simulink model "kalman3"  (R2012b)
settings: Solver=ode45  StartTime=0.0  StopTime=50.0  RelTol=1e-3
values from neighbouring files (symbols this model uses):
  A1 = 0.02    [fuellstnd_1.m]    (also in fuellstnd_2.m; fuellstnd_21.m; fuellstnd_3.m; fuellstnd_31.m)
  A2 = A1    (= 0.02)    [fuellstnd_1.m]    (also in fuellstnd_2.m; fuellstnd_21.m; fuellstnd_3.m; fuellstnd_31.m)
  B1 = sys1.b    [kalman_11.m]    (also in kalman_12.m; kalman_13.m; kalman_2.m; kalman_3.m)
  B2 = sys2.b    [kalman_2.m]    (also in kalman_3.m)
  C1 = sys1.c    [kalman_11.m]    (also in kalman_12.m; kalman_13.m; kalman_2.m; kalman_3.m)
  C2 = sys2.c    [kalman_2.m]    (also in kalman_3.m; feder_masse_1.m = [0 0 1 0]; feder_masse_13.m = [0 0 1 0]; feder_masse_14.m = [0 0 1 0])
  dt = 0.01    [aktiv_tilger_1.m]    (also in aktiv_tilger_12.m; aktiv_tilger_2.m; beobachter_1.m; beobachter_2.m)
  Kest = kalman(P,1,0.01),    [LQG_1.m]    (also in ss_zwei_eing_1.m = kalman(sys2, Q, R))
  ki = -Kn(n+1)    [beobachter_2.m]    (also in beobachter_22.m; kalman_12.m = -Kn(3); kalman_13.m = -Kn(4); kalman_d1.m = -Kn(4))
  Kr = 2000    [aktiv_tilger_2.m]    (also in beobachter_22.m = 5; fuellstnd_3.m = 10,; fuellstnd_31.m = 10,; kalman_12.m = Kn(1:2))
  vnd = 1e-4    (= 0.0001)    [kalman_1.m]    (also in kalman_10.m; kalman_11.m; kalman_12.m; kalman_13.m = 0.01)
  vny = 1e-6    (= 1e-06)    [kalman_1.m]    (also in kalman_10.m; kalman_11.m = ', num2str(vny),' )']); kalman_12.m = ', num2str(vny),' )']); kalman_13.m = ', num2str(vny),' )']))

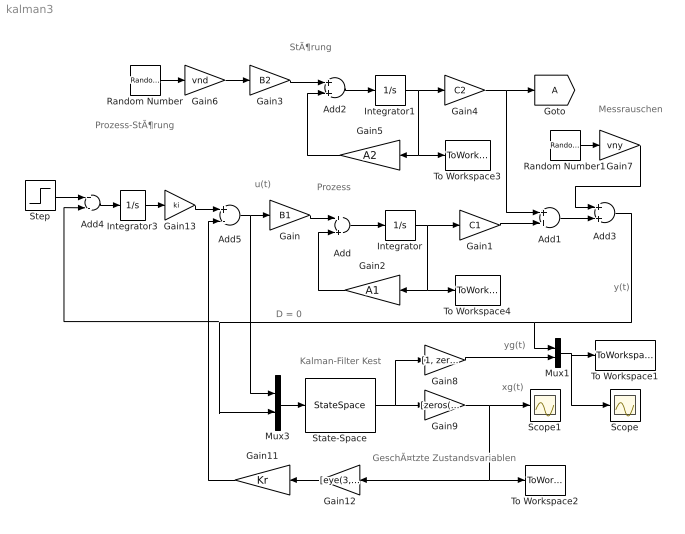
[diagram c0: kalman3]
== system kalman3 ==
  note: StÃ¶rung
  note: Prozess
  note: Prozess-StÃ¶rung
  note: Messrauschen
  note: xg(t)
  note: y(t)
  note: u(t)
  note: D = 0
  note: Kalman-Filter Kest
  note: yg(t)
  note: GeschÃ¤tzte Zustandsvariablen
  Add{,1..3} (4 alike) : Sum
  Add4 : Sum  Inputs=+-
  Add5 : Sum  Inputs=+-
  Gain : Gain  Gain=B1  Multiplication=Matrix(K*u)
  Gain1 : Gain  Gain=C1  Multiplication=Matrix(K*u)
  Gain11 : Gain  Gain=Kr  Multiplication=Matrix(K*u)
  Gain12 : Gain  Gain=[eye(3,3), zeros(3,3)]  Multiplication=Matrix(K*u)
  Gain13 : Gain  Gain=ki
  Gain2 : Gain  Gain=A1  Multiplication=Matrix(K*u)
  Gain3 : Gain  Gain=B2  Multiplication=Matrix(K*u)
  Gain4 : Gain  Gain=C2  Multiplication=Matrix(K*u)
  Gain5 : Gain  Gain=A2  Multiplication=Matrix(K*u)
  Gain6 : Gain  Gain=vnd
  Gain7 : Gain  Gain=vny
  Gain8 : Gain  Gain=[1, zeros(1,6)]  Multiplication=Matrix(K*u)
  Gain9 : Gain  Gain=[zeros(6,1),eye(6,6)]  Multiplication=Matrix(K*u)
  Integrator : Integrator
  Integrator1 : Integrator
  Integrator3 : Integrator
  Mux1 : Mux  Inputs=2
  Mux3 : Mux  Inputs=2
  Random Number : RandomNumber  SampleTime=dt*10
  Random Number1 : RandomNumber  Seed=18967  SampleTime=dt*10
  Scope : Scope
  Scope1 : Scope
  State-Space : StateSpace  A=Kest.a  B=Kest.b  C=Kest.c  D=Kest.d
  Step : Step  SampleTime=0
  To Workspace1 : ToWorkspace  VariableName=y1  SaveFormat=Structure With Time
  To Workspace2 : ToWorkspace  VariableName=y  SaveFormat=Structure With Time
  To Workspace3 : ToWorkspace  VariableName=y2  SaveFormat=Structure With Time
  To Workspace4 : ToWorkspace  VariableName=y3  SaveFormat=Structure With Time
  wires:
  Gain/1 -> Add/1
  Add/1 -> Integrator/1
  Integrator/1 -> To Workspace4/1, Gain2/1, Gain1/1
  Gain2/1 -> Add/2
  Gain6/1 -> Gain3/1
  Gain3/1 -> Add2/1
  Add2/1 -> Integrator1/1
  Integrator1/1 -> Gain4/1, To Workspace3/1, Gain5/1
  Gain5/1 -> Add2/2
  Random Number/1 -> Gain6/1
  Random Number1/1 -> Gain7/1
  Gain9/1 -> Scope1/1, To Workspace2/1, Gain12/1
  State-Space/1 -> Gain8/1, Gain9/1
  Add1/1 -> Add3/2
  Mux3/1 -> State-Space/1
  Gain7/1 -> Add3/1
  Mux1/1 -> Scope/1, To Workspace1/1
  Gain1/1 -> Add1/2
  Step/1 -> Add4/1
  Add5/1 -> Gain/1, Mux3/1
  Gain11/1 -> Add5/2
  Gain12/1 -> Gain11/1
  Gain8/1 -> Mux1/2
  Gain4/1 -> [A], Add1/1
  Add3/1 -> Mux1/1, Mux3/2, Add4/2
  Integrator3/1 -> Gain13/1
  Add4/1 -> Integrator3/1
  Gain13/1 -> Add5/1
